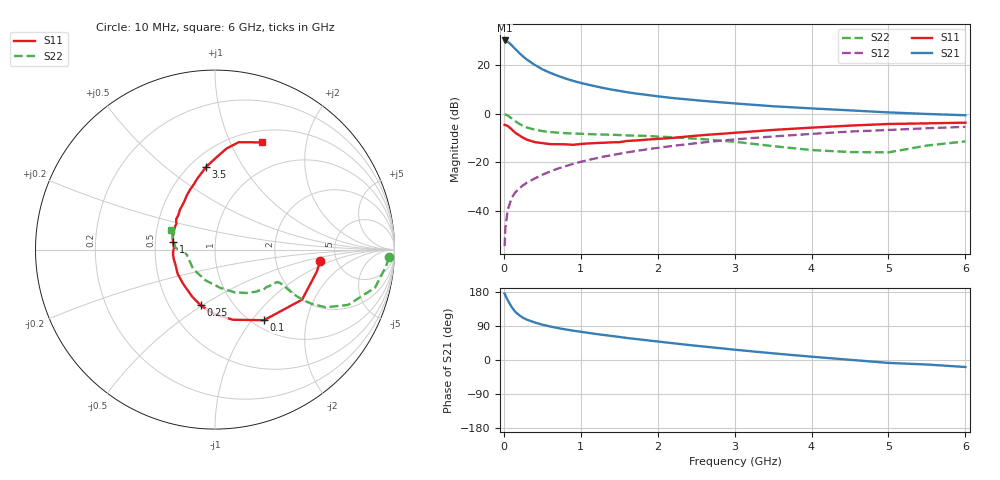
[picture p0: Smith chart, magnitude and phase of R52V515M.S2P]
! SIEMENS Small Signal Semiconductors
! BFR183
! Si NPN RF Bipolar Junction Transistor in SOT23
! VCE = 2.5 V  IC = 15 mA
! Common Emitter S-Parameters:  May  1996
# GHz  S  MA  R  50
!  f  S11  S21  S12  S22
! GHz  MAG  ANG  MAG  ANG  MAG  ANG  MAG  ANG
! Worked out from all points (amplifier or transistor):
!   36 points, 10 MHz to 6 GHz, reference 50 ohm
!   highest |S21| = 30.0 dB at 10 MHz (marker M1)
!   |S21| within 3 dB of that: start of sweep to 133.3 MHz
!   unconditionally stable (mu >= 1): 615.6 MHz to 2.403 GHz
!   at 250 MHz: K = 0.75, MSG = 26.5 dB, |S12| = -29.4 dB
!   at 1.4 GHz: K = 1.05, MAG = 12.1 dB, |S12| = -17.1 dB
!   at 6 GHz: K = 0.90, MSG = 2.4 dB, |S12| = -5.4 dB
!   S11 on the Smith chart (normalised r, x): 10 MHz: 3.72, -0.75; 100 MHz: 1.13, -1.15; 250 MHz: 0.71, -0.49; 1 GHz: 0.62, +0.06; 3.5 GHz: 0.60, +0.70; 6 GHz: 0.64, +1.33
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0.01  0.5902 -6.4  31.79 175.3  0.0019 93.4  0.9694 -2.6
0.02  0.58 -12.3  31.61 170.5  0.0045 80.7  0.9573 -5.6
0.05  0.5596 -29.9  30.01 157.8  0.0104 77.7  0.9161 -13.4
0.1  0.4788 -55.2  25.57 140.3  0.0184 70.5  0.8026 -22.6
0.15  0.4037 -75.6  21.11 127.0  0.0244 66.8  0.6961 -27.5
0.2  0.3582 -91.1  17.63 118.2  0.0292 65.7  0.6181 -29.3
0.25  0.3205 -104.5  14.9 111.4  0.0337 65.1  0.5602 -29.8
0.3  0.2916 -115.8  12.88 106.3  0.0382 66.3  0.5199 -29.7
0.4  0.2606 -133.0  10.05 99.2  0.0464 67.2  0.4683 -28.7
0.5  0.248 -147.2  8.154 93.3  0.0556 68.3  0.4382 -27.8
0.6  0.2365 -157.9  6.909 88.5  0.0648 68.8  0.4203 -27.3
0.7  0.2358 -168.5  5.989 84.4  0.0741 69.4  0.4071 -27.2
0.8  0.2345 -176.5  5.264 80.8  0.083 69.0  0.3974 -27.3
1  0.2382 169.4  4.271 74.4  0.1024 68.4  0.3859 -28.3
1.1  0.2445 164.7  3.921 71.6  0.1117 68.2  0.3806 -29.5
1.3  0.2524 154.4  3.344 66.0  0.1312 66.6  0.3712 -31.4
1.6  0.2745 142.0  2.759 58.1  0.1597 64.1  0.3568 -35.5
2.2  0.3177 122.7  2.086 44.2  0.2179 58.3  0.3275 -45.7
3.5  0.4627 96.2  1.418 17.6  0.3395 42.3  0.2152 -82.2
4.5  0.5676 83.4  1.166 0.5  0.4284 29.7  0.1626 -138.7
5.5  0.6316 71.2  0.984 -11.9  0.5015 17.8  0.2212 177.3
6  0.6521 66.3  0.927 -18.5  0.5352 10.1  0.2693 155.5
